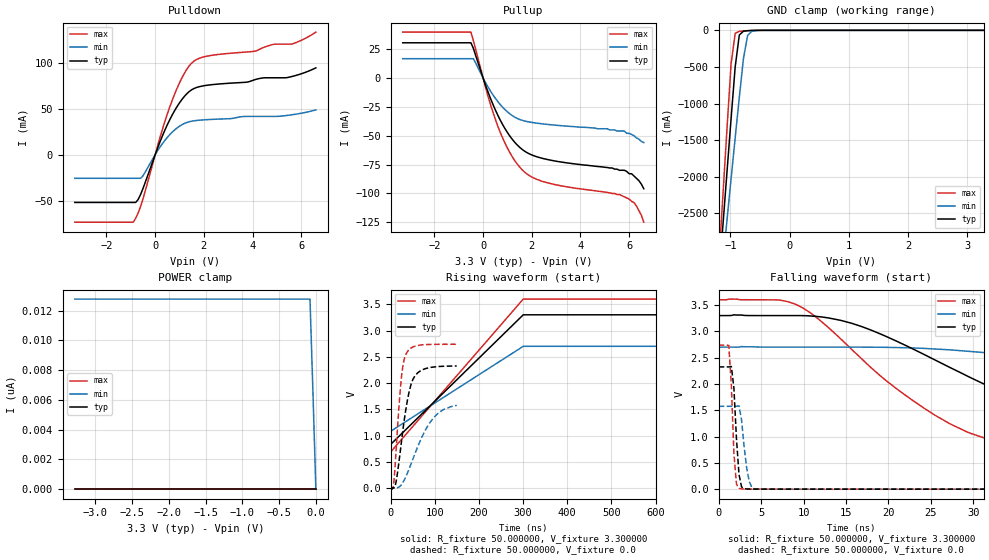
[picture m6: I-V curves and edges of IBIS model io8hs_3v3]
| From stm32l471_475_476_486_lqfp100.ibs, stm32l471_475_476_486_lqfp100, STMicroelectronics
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|   Model io8hs_3v3
[Model]  io8hs_3v3
Model_type I/O
Polarity   Non-Inverting
Enable   Active-Low
Vinl =   0.990000V
Vinh =   2.310000V
Vmeas =  1.650000V
Cref =   100.000000nF
Rref =   1.000000k
Vref =   3.300000V
C_comp   2.267200pF   2.233100pF   2.322300pF
[Temperature Range]   25.000000   0.125000k   -40.000000
[Pullup Reference]   3.300000V   2.700000V   3.600000V
[Pulldown Reference]   0.0V   0.0V   0.0V
[POWER Clamp Reference]   3.300000V   2.700000V   3.600000V
[GND Clamp Reference]   0.0V   0.0V   0.0V
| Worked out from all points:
|   slope of the pulldown table from 0 to 0.495 V, typ, clamps not added: 15.3 ohm
|   slope of the pullup table from 0 to 0.495 V, typ, clamps not added: 18.1 ohm
|   GND clamp passes 1 mA (typ) near -0.58 V on its own axis
|   rising waveform, R_fixture 50.000000, V_fixture 3.300000: 20-80 % time 180ns typ, 180ns min, 180ns max; typ from 0.831 V to 3.3 V
|   rising waveform, R_fixture 50.000000, V_fixture 0.0: 20-80 % time 24.3ns typ, 50.9ns min, 14.6ns max; typ from 0 V to 2.33 V
|   falling waveform, R_fixture 50.000000, V_fixture 3.300000: 20-80 % time 21ns typ, 41.5ns min, 13.6ns max; typ from 3.3 V to 0.831 V
|   falling waveform, R_fixture 50.000000, V_fixture 0.0: 20-80 % time 499ps typ, 675ps min, 456ps max; typ from 2.33 V to 0 V
[Pulldown]
|Voltage   I(typ)   I(min)   I(max)
-3.3V     -51.87mA   -25.68mA   -73.32mA
-900mV    -51.87mA   -25.68mA   -73.32mA
-700mV    -48.68mA   -25.68mA   -63.27mA
-500mV    -36.68mA   -22.92mA   -47.9mA
200mV     14.09mA    8.363mA    18.97mA
700mV     43.2mA     24.54mA    59.15mA
1.2V      63.38mA    34mA       88.53mA
1.6V      72.01mA    36.89mA    101.8mA
4.1V      81.58mA    41.61mA    112.4mA
4.9V      83.61mA    41.61mA    120.1mA
5.6V      84.89mA    43.33mA    120.1mA
6.6V      94.39mA    48.68mA    133.3mA
[Pullup]
|Voltage   I(typ)   I(min)   I(max)
-3.3V     30.51mA    16.73mA    39.79mA
-500mV    30.51mA    16.73mA    39.79mA
-400mV    25.73mA    16.73mA    32.44mA
200mV     -11.99mA   -7.69mA    -15.6mA
500mV     -27.53mA   -17.49mA   -35.6mA
1V        -47.29mA   -29.38mA   -60.81mA
1.5V      -60.05mA   -35.95mA   -77.15mA
1.9V      -65.77mA   -38.13mA   -84.64mA
2.6V      -70.47mA   -40.14mA   -90.6mA
5.6V      -80mA      -46mA      -101mA
6.2V      -85mA      -50mA      -108mA
6.6V      -96mA      -56mA      -125mA
[GND_clamp]
|Voltage   I(typ)   I(min)   I(max)
-3.3V     -9.456A    -9.706A    -9.779A
-1.2V     -3.441A    -3.76A     -3.218A
-1.13V    -2.694A    -3.182A    -2.288A
-1.06V    -1.951A    -2.607A    -1.365A
-990mV    -1.216A    -2.035A    -464.9mA
-920mV    -500mA     -1.468A    -40.15mA
-850mV    -63.51mA   -913mA     -13.79mA
-780mV    -11.84mA   -384.3mA   -8.858mA
-710mV    -4.78mA    -70.26mA   -5.228mA
-640mV    -2.25mA    -14.29mA   -2.447mA
-430mV    -27.1uA    -149uA     -11.19uA
3.28V     0A         0A         0A
[POWER_clamp]
|Voltage   I(typ)   I(min)   I(max)
-3.28V    0A         12.77nA    0A
-80mV     0A         12.77nA    0A
-40mV     0A         6.549nA    0A
0V        0A         0A         0A
[Ramp]
| variable   typ   min   max
dV/dt_r  1.39476/24.30683n   0.94506/54.41207n   1.64316/14.55319n
dV/dt_f  1.48126/21.06482n   0.97098/44.57739n   1.74767/13.63828n
R_load = 50.000000
[Rising Waveform]
R_fixture= 50.000000
V_fixture= 3.300000
V_fixture_min= 2.700000
V_fixture_max= 3.600000
|time   V(typ)   V(min)   V(max)
0s        831.2mV    1.082V     687.2mV
300.3ns   3.3V       2.7V       3.6V
600.6ns   3.3V       2.7V       3.6V
29.73us   3.3V       2.7V       3.6V
[Rising Waveform]
R_fixture= 50.000000
V_fixture= 0.0
V_fixture_min= 0.0
V_fixture_max= 0.0
|time   V(typ)   V(min)   V(max)
0s        2.592nV    41.12nV    2.445nV
6.006ns   -212.3uV   -165.9uV   34.14mV
11.71ns   98.71mV    239uV      645.5mV
18.62ns   491.4mV    17.55mV    1.541V
24.62ns   899.6mV    66.19mV    2.13V
35.44ns   1.551V     236.3mV    2.563V
46.55ns   1.987V     468.9mV    2.668V
61.86ns   2.2V       800.2mV    2.717V
96.7ns    2.305V     1.334V     2.736V
149.5ns   2.325V     1.575V     2.739V
[Falling Waveform]
R_fixture= 50.000000
V_fixture= 3.300000
V_fixture_min= 2.700000
V_fixture_max= 3.600000
|time   V(typ)   V(min)   V(max)
0s        3.3V       2.7V       3.6V
9.309ns   3.3V       2.7V       3.497V
15.92ns   3.141V     2.7V       2.62V
25.53ns   2.453V     2.664V     1.402V
29.73ns   2.116V     2.617V     1.059V
35.14ns   1.728V     2.529V     872.5mV
45.65ns   1.184V     2.294V     770mV
56.76ns   995.6mV    2.009V     727.7mV
91.89ns   863.6mV    1.303V     693.4mV
149.5ns   831.2mV    1.082V     687.2mV
[Falling Waveform]
R_fixture= 50.000000
V_fixture= 0.0
V_fixture_min= 0.0
V_fixture_max= 0.0
|time   V(typ)   V(min)   V(max)
0s        2.325V     1.575V     2.739V
1.201ns   2.325V     1.575V     2.732V
1.502ns   2.332V     1.575V     1.968V
1.802ns   1.923V     1.575V     679.7mV
2.102ns   963.4mV    1.576V     97.58mV
2.402ns   277.6mV    1.585V     16.45mV
2.703ns   43.49mV    1.314V     4.545mV
3.604ns   2.411mV    148.4mV    1.95mV
4.505ns   1.415mV    3.366mV    1.522mV
149.5ns   2.592nV    41.12nV    2.445nV
